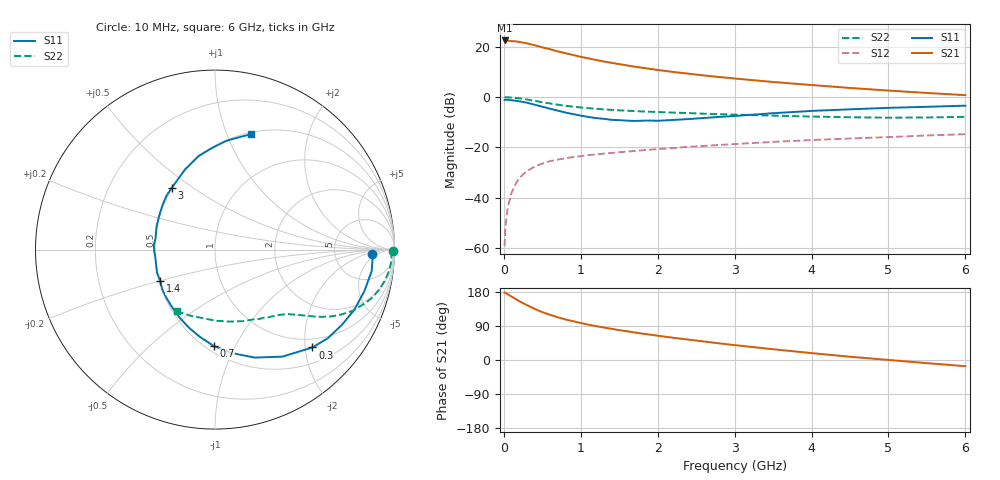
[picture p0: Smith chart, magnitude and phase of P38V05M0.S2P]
! SIEMENS Small Signal Semiconductors
! BFP181
! Si NPN RF Bipolar Junction Transistor in SOT143
! VCE = 8 V  IC = 5 mA
! Common Emitter S-Parameters:  March  1996
# GHz  S  MA  R  50
!  f  S11  S21  S12  S22
! GHz  MAG  ANG  MAG  ANG  MAG  ANG  MAG  ANG
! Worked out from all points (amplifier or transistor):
!   36 points, 10 MHz to 6 GHz, reference 50 ohm
!   highest |S21| = 22.4 dB at 10 MHz (marker M1)
!   |S21| within 3 dB of that: start of sweep to 535.7 MHz
!   unconditionally stable (mu >= 1): 1.86 GHz to end of sweep
!   at 250 MHz: K = 0.20, MSG = 26.1 dB, |S12| = -30.8 dB
!   at 1.4 GHz: K = 0.87, MSG = 17.9 dB, |S12| = -22.2 dB
!   at 6 GHz: K = 1.06, MAG = 6.2 dB, |S12| = -14.8 dB
!   lowest NFmin = 1.55 dB at 450 MHz
!   S11 on the Smith chart (normalised r, x): 10 MHz: 15, -3; 300 MHz: 0.81, -2.16; 700 MHz: 0.55, -0.82; 1.4 GHz: 0.51, -0.20; 3 GHz: 0.50, +0.42; 6 GHz: 0.52, +1.22
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0.01  0.8774 -1.7  13.22 178.0  0.0011 91.9  0.9895 -0.6
0.02  0.8793 -3.3  13.22 177.5  0.0027 76.1  0.983 -1.4
0.05  0.8813 -7.8  13.13 173.5  0.0064 85.1  0.986 -3.6
0.15  0.8451 -23.6  12.69 161.2  0.0185 76.5  0.9612 -10.5
0.2  0.8213 -30.9  12.39 155.4  0.0246 72.7  0.9413 -13.7
0.25  0.7994 -38.1  11.95 149.8  0.029 69.5  0.9177 -16.8
0.3  0.7695 -45.1  11.59 144.8  0.0339 65.8  0.8922 -19.3
0.4  0.7047 -57.8  10.64 134.8  0.0416 60.2  0.8391 -24.0
0.5  0.6416 -69.7  9.647 126.4  0.0479 55.4  0.7897 -27.3
0.6  0.5856 -80.4  8.871 119.2  0.0536 52.0  0.7437 -30.1
0.7  0.5368 -90.8  8.023 112.8  0.0572 48.9  0.7033 -32.2
0.8  0.4916 -100.2  7.41 107.1  0.0608 46.8  0.6705 -33.8
0.9  0.4586 -108.5  6.8 102.3  0.0644 44.9  0.6419 -35.2
1.1  0.4018 -126.0  5.841 93.2  0.0704 42.6  0.5998 -37.5
1.4  0.3519 -150.2  4.764 82.3  0.0777 40.2  0.5557 -40.5
1.8  0.3387 -178.7  3.799 69.6  0.0876 38.4  0.5175 -44.5
2.2  0.3504 158.3  3.143 58.7  0.0971 36.9  0.4902 -49.3
3  0.4204 124.8  2.33 39.3  0.1166 32.8  0.4459 -60.5
3.5  0.4769 110.5  1.985 28.4  0.1287 29.9  0.4275 -68.9
4.5  0.5695 91.1  1.511 8.6  0.1504 23.2  0.3967 -88.9
5.5  0.6387 78.2  1.203 -8.3  0.1724 17.5  0.3929 -110.3
6  0.6731 72.7  1.088 -16.4  0.183 13.9  0.4039 -121.4
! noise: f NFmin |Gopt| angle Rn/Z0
0.45  1.55  0.48  17  0.36
0.9  1.65  0.4  35  0.34
1.8  2  0.18  88  0.34
